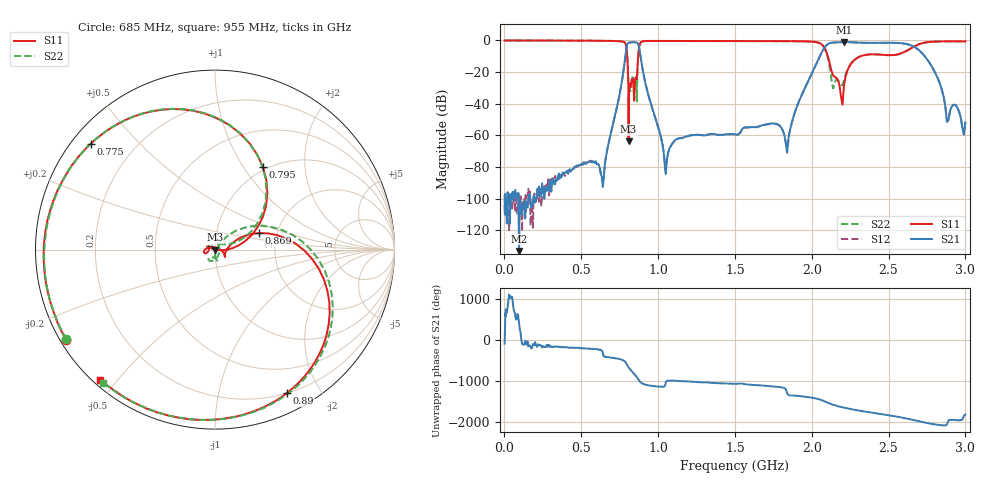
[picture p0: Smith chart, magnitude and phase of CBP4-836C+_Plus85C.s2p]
! Mini-Circuits
! S2P DATA File Format
! Type: BAND PASS FILTER
! Model: CBP4-836C+
! All S Parameters are in dB deg format
! TEST CONDITIONS: INPUT POWER = 0 dBm @ Temperature = +85deg C
! 636 Frequency points
# MHz S DB R 50
!FREQMAG(S11)PHS(S11)MAG(S21)PHS(S21)MAG(S12)PHS(S12)MAG(S22)PHS(S22)
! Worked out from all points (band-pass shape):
!   636 points, 1 MHz to 3 GHz, reference 50 ohm
!   highest |S21| = -1.04 dB at 2.21 GHz (marker M1); lowest = -133.1 dB at 95 MHz (marker M2)
!   |S21| within 3 dB of the highest: 795.4 MHz to 875.4 MHz (80 MHz wide, 9.58 % of centre); 2.086 GHz to 2.667 GHz (580.8 MHz wide, 24.4 % of centre)
!   lowest |S11| = -63.7 dB at 808 MHz (marker M3), VSWR 1.00, Z = 50 + j0.0513 ohm
!   |S11| at or under -10 dB: 799.1 MHz to 870.2 MHz (71.1 MHz wide, 8.52 % of centre); 2.105 GHz to 2.318 GHz (213.2 MHz wide, 9.64 % of centre)
!   |S22| runs from -38.6 to 0.0 dB; largest |S21 - S12| = 0.016
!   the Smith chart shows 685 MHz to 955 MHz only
!   S11 on the Smith chart (normalised r, x): 685 MHz: 0.02, -0.28; 775 MHz: 0.05, +0.37; 795 MHz: 0.95, +1.23; 869 MHz: 1.62, +0.32; 890 MHz: 0.20, -1.61; 955 MHz: 0.02, -0.45
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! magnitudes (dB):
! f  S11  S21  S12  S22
! 1 MHz  0.0  -98.1  -104.0  0.0
! 95 MHz  0.0  -133.1  -96.5  0.0
! 505 MHz  -0.1  -78.6  -77.8  -0.1
! 635 MHz  -0.2  -86.5  -88.8  -0.2
! 685 MHz  -0.3  -61.7  -61.5  -0.3
! 775 MHz  -0.8  -18.9  -18.9  -0.8
! 795 MHz  -5.5  -4.3  -4.2  -5.4
! 808 MHz  -63.7  -1.5  -1.4  -27.5
! 861 MHz  -24.4  -1.3  -1.3  -37.4
! 869 MHz  -11.6  -2.0  -2.0  -12.2
! 890 MHz  -1.0  -12.8  -12.8  -1.0
! 955 MHz  -0.3  -40.6  -40.6  -0.3
! 1.005 GHz  -0.3  -56.3  -56.2  -0.3
! 1.05 GHz  -0.3  -84.4  -82.4  -0.3
! 1.505 GHz  -0.4  -59.5  -59.4  -0.4
! 1.84 GHz  -0.4  -70.5  -71.0  -0.5
! 2.01 GHz  -0.8  -18.9  -18.9  -0.9
! 2.21 GHz  -28.2  -1.0  -1.1  -25.2
! 2.3 GHz  -10.8  -1.3  -1.3  -10.8
! 2.51 GHz  -9.3  -1.4  -1.5  -9.3
! 2.72 GHz  -1.7  -8.2  -8.3  -1.8
! 3 GHz  -0.6  -51.8  -51.9  -0.7
